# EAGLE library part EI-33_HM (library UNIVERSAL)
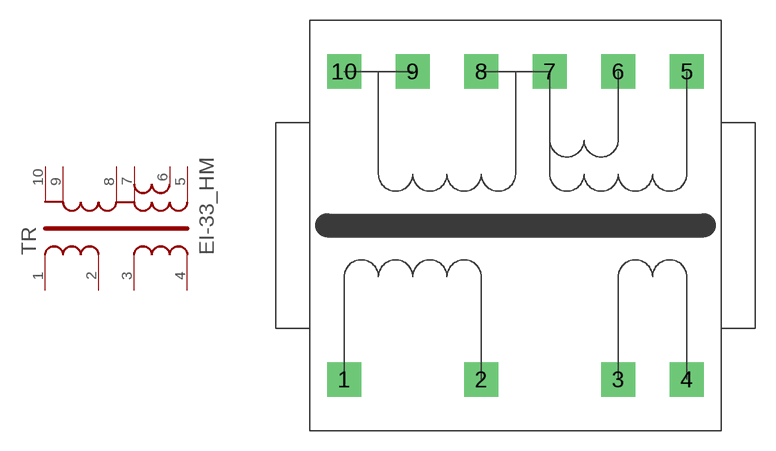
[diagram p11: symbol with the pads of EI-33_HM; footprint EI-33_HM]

Designator prefix TR

## EI-33_HM  [EI-33_HM]
1  1
2  2
3  3
4  4
5  5
6  6
7  7
8  8
9  9
10  10

## Footprint EI-33_HM (pad centres in mm)
drill 0.813 pad 2.54 square: 1 0,0; 2 10.16,0; 3 20.32,0; 4 25.4,0; 5 25.4,22.86; 6 20.32,22.86; 7 15.24,22.86; 8 10.16,22.86; 9 5.08,22.86; 10 0,22.86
